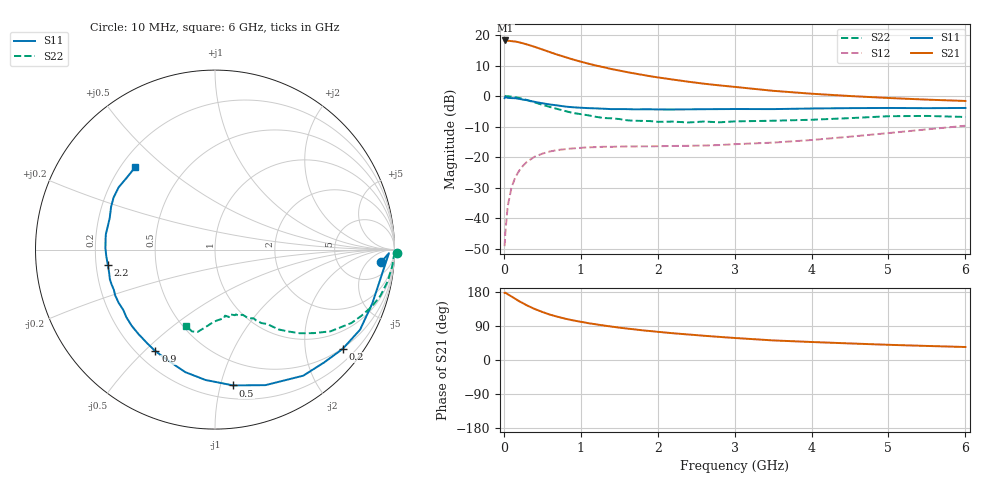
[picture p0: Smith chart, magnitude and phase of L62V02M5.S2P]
!  INFINEON TECHNOLOGIES Small Signal Semiconductors
! BFR380L3 , Si-NPN RF-Transistor in TSLP-3-1
!  Vce=2 V,  Ic=2.5 mA
! Common Emitter S-Parameters:  07. March 2005
#  GHz  S  MA  R  50
! f  S11  S21  S12  S22
! GHz  Mag  Ang  Mag  Ang  Mag  Ang  Mag  Ang
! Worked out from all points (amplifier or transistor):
!   36 points, 10 MHz to 6 GHz, reference 50 ohm
!   highest |S21| = 18.2 dB at 20 MHz (marker M1)
!   |S21| within 3 dB of that: start of sweep to 505.7 MHz
!   unconditionally stable (mu >= 1): 2.695 GHz to 4.693 GHz
!   at 250 MHz: K = 0.10, MSG = 20.0 dB, |S12| = -22.8 dB
!   at 1.4 GHz: K = 0.60, MSG = 12.7 dB, |S12| = -16.6 dB
!   at 6 GHz: K = 0.92, MSG = 4.1 dB, |S12| = -9.7 dB
!   S11 on the Smith chart (normalised r, x): 10 MHz: 13, -13; 200 MHz: 0.48, -2.84; 500 MHz: 0.30, -1.10; 900 MHz: 0.27, -0.54; 2.2 GHz: 0.25, -0.07; 6 GHz: 0.26, +0.40
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0.01  0.9263 -4.4  8.102 177.1  0.0035 87.7  1.014 -1.1
0.02  0.9691 -1.2  8.134 177.7  0.0059 92.3  0.9964 -2.3
0.05  0.9365 -9.8  8.064 173.7  0.0157 86.6  0.9922 -5.2
0.1  0.9265 -18.9  7.927 167.6  0.0321 79.9  0.9781 -10.4
0.15  0.9233 -28.9  7.811 161.3  0.0473 74.4  0.9575 -15.5
0.2  0.901 -37.9  7.573 155.0  0.0603 70.4  0.9304 -19.9
0.3  0.8575 -55.0  6.999 144.1  0.084 61.4  0.8628 -28.3
0.4  0.8057 -69.6  6.402 134.7  0.1018 54.0  0.7881 -35.3
0.5  0.7634 -82.4  5.792 126.8  0.1141 48.5  0.7209 -40.2
0.6  0.7282 -94.2  5.232 119.7  0.1242 44.0  0.6638 -44.6
0.7  0.7026 -103.6  4.746 114.1  0.1311 40.7  0.6132 -48.1
0.8  0.6732 -112.0  4.337 108.9  0.1354 38.0  0.5683 -51.5
0.9  0.6561 -120.4  3.968 104.5  0.1394 35.8  0.5286 -53.6
1.1  0.635 -132.1  3.392 97.1  0.1449 33.4  0.4843 -57.7
1.5  0.6132 -151.1  2.619 85.4  0.1492 31.5  0.4212 -64.4
1.9  0.6086 -164.3  2.116 76.4  0.1506 32.4  0.3902 -70.7
2.2  0.6031 -171.9  1.862 70.6  0.1527 34.6  0.3822 -73.1
2.8  0.6121 175.1  1.498 61.0  0.1579 41.0  0.3722 -81.4
3.5  0.6123 163.4  1.22 51.7  0.1732 48.3  0.3952 -88.5
4.5  0.6352 152.8  1.002 43.7  0.2167 58.9  0.436 -97.1
5.5  0.6342 140.8  0.875 37.1  0.2852 63.0  0.4736 -105.8
6  0.6394 134.0  0.832 34.3  0.3271 62.8  0.455 -110.5
